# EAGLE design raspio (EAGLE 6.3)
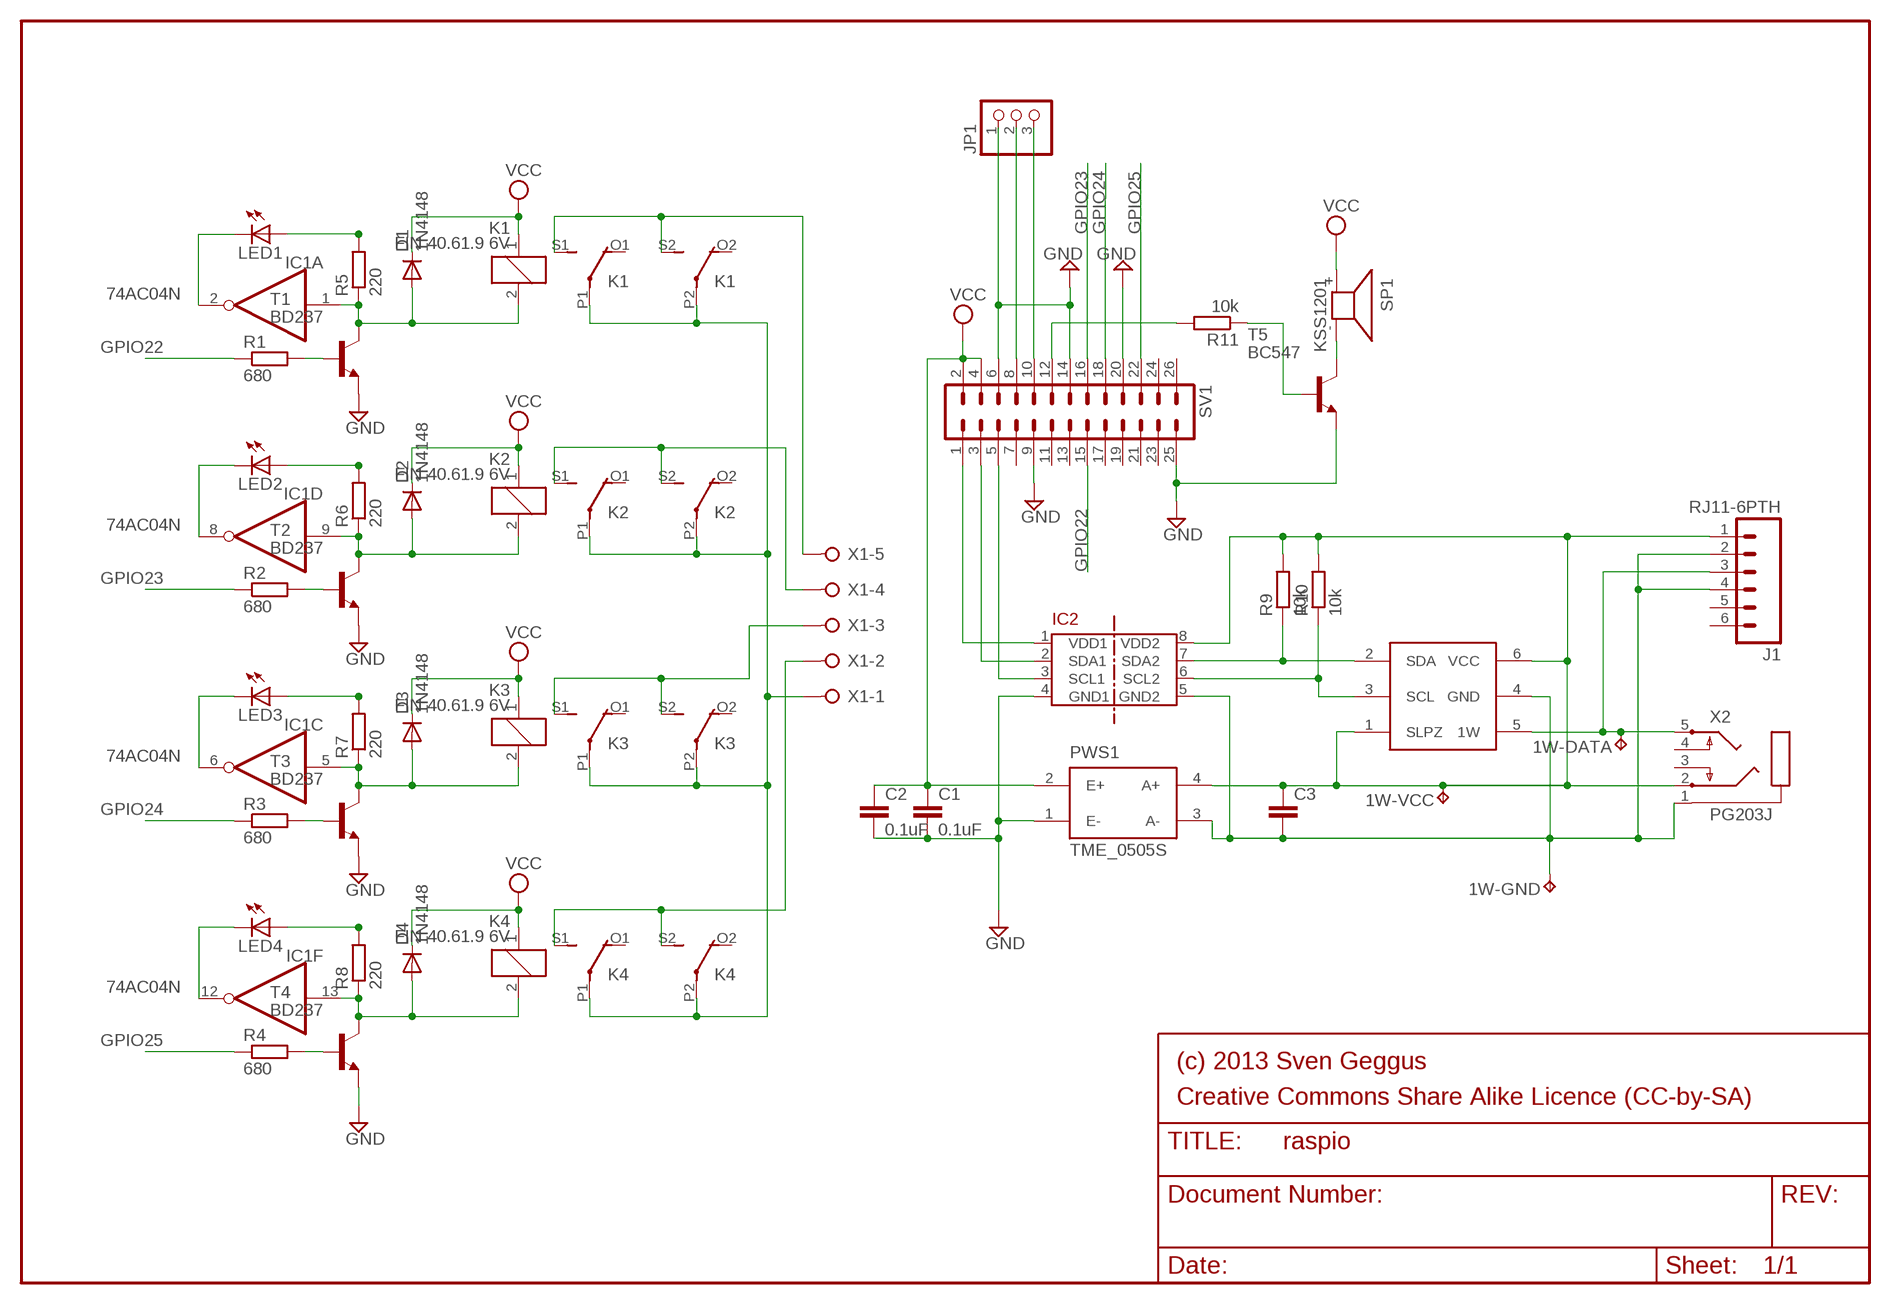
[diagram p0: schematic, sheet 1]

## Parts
1W-DATA  TPPAD1-13  [P1-13]
1W-GND  TPPAD1-13  [P1-13]
1W-VCC  TPPAD1-13  [P1-13]
C1  0.1uF  C-EU025-024X044  [C025-024X044]
C2  0.1uF  C-EU025-024X044  [C025-024X044]
C3  C-EU025-024X044  [C025-024X044]
D1  1N4148  [DO35-10]
D2  1N4148  [DO35-10]
D3  1N4148  [DO35-10]
D4  1N4148  [DO35-10]
IC1  74AC04N  [DIL14]
IC2  ADUM1250  [SO08]
IC3  DS2483  [TSOT23]
J1  RJ11-6PTH  [RJ11-6]
JP1  PINHD-1X3  [1X03]
K1  FIN 40.61.9 6V  4052  [F4052]
K2  FIN 40.61.9 6V  4052  [F4052]
K3  FIN 40.61.9 6V  4052  [F4052]
K4  FIN 40.61.9 6V  4052  [F4052]
LED1  LED5MM  [LED5MM]
LED2  LED5MM  [LED5MM]
LED3  LED5MM  [LED5MM]
LED4  LED5MM  [LED5MM]
PWS1  TME_0505S  [TMEXXXXS]
R1  680  R-EU_0207/10  [0207/10]
R2  680  R-EU_0207/10  [0207/10]
R3  680  R-EU_0207/10  [0207/10]
R4  680  R-EU_0207/10  [0207/10]
R5  220  R-EU_0207/10  [0207/10]
R6  220  R-EU_0207/10  [0207/10]
R7  220  R-EU_0207/10  [0207/10]
R8  220  R-EU_0207/10  [0207/10]
R9  10k  R-EU_0207/10  [0207/10]
R10  10k  R-EU_0207/10  [0207/10]
R11  10k  R-EU_0207/10  [0207/10]
SP1  KSS1201  [KSS1201]
SV1  ML26  [ML26]
T1  BD237  [TO126V]
T2  BD237  [TO126V]
T3  BD237  [TO126V]
T4  BD237  [TO126V]
T5  BC547  [TO92]
X1  W237-05P  [W237-5P]
X2  PG203J  [PG203J]

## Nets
GND: C1.2 C2.2 IC2.4(GND1) JP1.1 PWS1.1(E-) SV1.6 SV1.9 SV1.14 SV1.20 SV1.25 T1.1(E) T2.1(E) T3.1(E) T4.1(E) T5.1(E)
GPIO22: R1.1 SV1.15
GPIO23: R2.1 SV1.16
GPIO24: R3.1 SV1.18
GPIO25: R4.1 SV1.22
L: K3.S1(2:S) K3.S2(3:S) X1.3
N$1: K1.P1(2:P) K1.P2(3:P) K2.P1(2:P) K2.P2(3:P) K3.P1(2:P) K3.P2(3:P) K4.P1(2:P) K4.P2(3:P) X1.1
N$2: R1.2 T1.3(B)
N$3: IC1.2(A:O) LED1.K(C)
N$4: D2.A IC1.9(D:I) K2.2 R6.1 T2.2(C)
N$5: R11.2 SV1.12
N$6: R11.1 T5.2(B)
N$7: R2.2 T2.3(B)
N$8: D3.A IC1.5(C:I) K3.2 R7.1 T3.2(C)
N$9: K1.S1(2:S) K1.S2(3:S) X1.5
N$10: K2.S1(2:S) K2.S2(3:S) X1.4
N$11: R3.2 T3.3(B)
N$12: D4.A IC1.13(F:I) K4.2 R8.1 T4.2(C)
N$13: K4.S1(2:S) K4.S2(3:S) X1.2
N$14: SP1.- T5.3(C)
N$15: R4.2 T4.3(B)
N$16: D1.A IC1.1(A:I) K1.2 R5.1 T1.2(C)
N$18: IC1.8(D:O) LED2.K(C)
N$19: IC1.6(C:O) LED3.K(C)
N$20: IC1.12(F:O) LED4.K(C)
N$21: LED1.A R5.2
N$22: LED2.A R6.2
N$23: LED3.A R7.2
N$24: LED4.A R8.2
OW: 1W-DATA.TP IC3.5(1W) J1.3 X2.5
OWGND: 1W-GND.TP C3.2 IC2.5(GND2) IC3.4(GND) J1.2 J1.4 PWS1.3(A-) X2.1
OWSCL: IC2.6(SCL2) IC3.3(SCL) R10.1
OWSDA: IC2.7(SDA2) IC3.2(SDA) R9.1
OWVCC: 1W-VCC.TP C3.1 IC2.8(VDD2) IC3.1(SLPZ) IC3.6(VCC) J1.1 PWS1.4(A+) R9.2 R10.2 X2.2
RXD: JP1.3 SV1.10
SCL: IC2.3(SCL1) SV1.5
SDA: IC2.2(SDA1) SV1.3
TXD: JP1.2 SV1.8
VCC: C1.1 C2.1 D1.C D2.C D3.C D4.C K1.1 K2.1 K3.1 K4.1 PWS1.2(E+) SP1.+ SV1.2 SV1.4
VDD: IC2.1(VDD1) SV1.1
Unconnected: IC1.3(B:I) IC1.4(B:O) IC1.10(E:O) IC1.11(E:I) J1.5 J1.6 K1.O1(2:O) K1.O2(3:O) K2.O1(2:O) K2.O2(3:O) K3.O1(2:O) K3.O2(3:O) K4.O1(2:O) K4.O2(3:O) SV1.7 SV1.11 SV1.13 SV1.17 SV1.19 SV1.21 SV1.23 SV1.24 SV1.26 X2.3 X2.4

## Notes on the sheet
- (c) 2013 Sven Geggus
- Creative Commons Share Alike Licence (CC-by-SA)

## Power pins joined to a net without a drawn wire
GND: IC1.7(P:GND)
VCC: IC1.14(P:VCC)

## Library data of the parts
1W-DATA 1W-GND 1W-VCC = testpad:TP: Test pad
C1-C3 = rcl:C-EU: CAPACITOR, European symbol
D1-D4 = diode:1N4148: DIODE
IC1 = 74xx-eu:74*04: Hex INVERTER
IC2 = Bus-isolators:ADUM1250
IC3 = ds2483:DS2483: Single-Channel 1-Wire Master with Adjustable Timing and Sleep Mode
J1 = SparkFun-Connectors:RJ11-6: RJ11 Jack Simple 6 pin RJ11 jack. Commonly found on CAT3 devices and Microchip programmers. SKU: PRT-00132
JP1 = pinhead:PINHD-1X3: PIN HEADER
K1-K4 = relay:4052: RELAY 2 x switch, Finder
LED1-LED4 = led:LED: LED
PWS1 = traco-electronic:TME_*S: DC/DC Konverter 1 Watt Source: http://www.tracopower.com/datasheet_g/tme-d.pdf; MPN: TME 0505S; OC_FARNELL: 1007538; OC_NEWARK: 51R5321
R1-R11 = resistor:R-EU_: RESISTOR, European symbol
SP1 = buzzer:KSS1201: SPEAKER; OC_FARNELL: unknown; OC_NEWARK: unknown
SV1 = con-ml:ML26: HARTING; OC_FARNELL: unknown; OC_NEWARK: unknown
T1-T4 = sven-misc:BD237: NPN Transistor
T5 = transistor:BC547: NPN TRANSISTOR
X1 = con-wago-508:W237-05P: WAGO SREW CLAMP; OC_FARNELL: unknown; OC_NEWARK: unknown
X2 = con-hirschmann:PG203J: MIC/HEADPHONE JACK KS-S stereo microphone/headphone jack PG203JN (Schukat); OC_FARNELL: unknown; OC_NEWARK: unknown

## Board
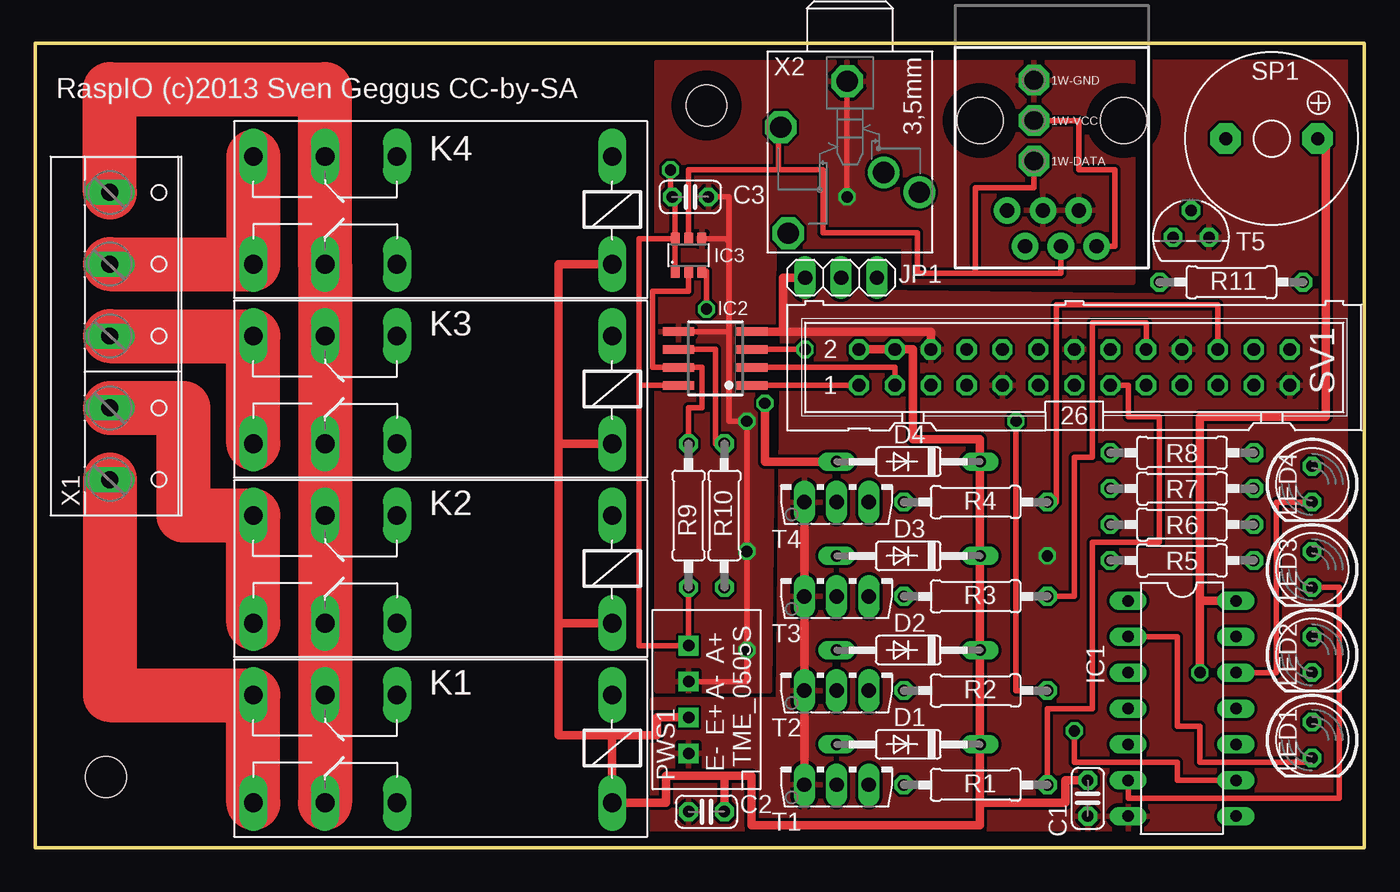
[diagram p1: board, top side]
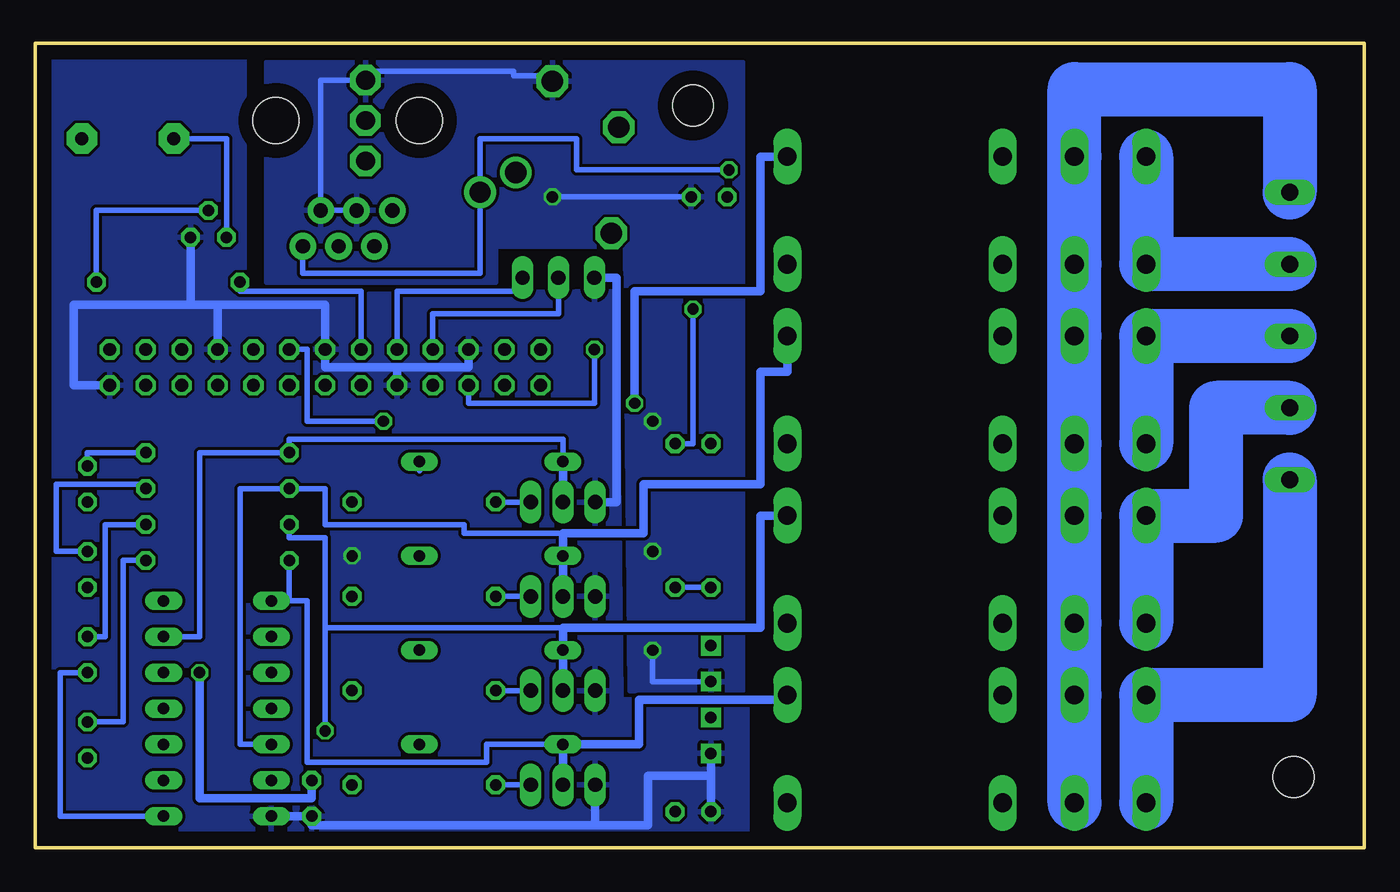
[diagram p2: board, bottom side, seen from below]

Size 94.05 x 56.92 mm. Coordinates in mm from the lower left corner, seen from the top.
Outline: 0,0 94.05,0 94.05,56.92 0,56.92 0,0
Copper layers (1*16): Top 0.035mm / dielectric 1.5mm / Bottom 0.035mm
Design rules "default": minimum track width 10mil, minimum drill 24mil, track to track 8mil, track to pad 8mil, pad to pad 8mil, via to via 8mil, smd to smd 8mil, copper to edge 40mil, drill to drill 8mil, minimum pad ring 10mil, minimum via ring 8mil, stop-mask expansion 4mil, vias tented up to drill 0mil, thermal gap 10mil
Holes 2.9 mm at 47.5,52.5 5,5

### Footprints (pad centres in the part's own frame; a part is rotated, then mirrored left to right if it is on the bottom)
P1-13 = drill 1.321 pad 2.159 octagon: TP 0,0
C025-024X044 = drill 0.813 octagon: 1 -1.27,0; 2 1.27,0
DO35-10 = drill 0.813 long: A 5.08,0; C -5.08,0
DIL14 = drill 0.813 long: 1 -7.62,-3.81; 2 -5.08,-3.81; 3 -2.54,-3.81; 4 0,-3.81; 5 2.54,-3.81; 6 5.08,-3.81; 7 7.62,-3.81; 8 7.62,3.81; 9 5.08,3.81; 10 2.54,3.81; 11 0,3.81; 12 -2.54,3.81; 13 -5.08,3.81; 14 -7.62,3.81
SO08 = smd 0.6 x 2.2: 1 -1.905,-2.6; 2 -0.635,-2.6; 3 0.635,-2.6; 4 1.905,-2.6; 5 1.905,2.6; 6 0.635,2.6; 7 -0.635,2.6; 8 -1.905,2.6
TSOT23 = smd 0.6 x 0.9: 1 -0.95,-1.15; 2 0,-1.15; 3 0.95,-1.15; 4 0.95,1.15; 5 0,1.15; 6 -0.95,1.15
RJ11-6 = drill 1.016 pad 1.88: 1 1.905,8.89; 2 3.175,6.35; 3 4.445,8.89; 4 5.715,6.35; 5 6.985,8.89; 6 8.255,6.35 | hole 3.251: 0,0; 10.16,0
1X03 = drill 1.016 long: 1 -2.54,0; 2 0,0; 3 2.54,0
F4052 = drill 1.321 long: 1 -3.81,3.81; 2 -3.81,-3.81; O1 11.43,-3.81; O2 11.43,3.81; P1 16.51,-3.81; P2 16.51,3.81; S1 21.59,-3.81; S2 21.59,3.81
LED5MM = drill 0.813 octagon: A -1.27,0; K 1.27,0
TMEXXXXS = drill 0.813 pad 1.397 square: 1 -3.81,1.27; 2 -1.27,1.27; 3 1.27,1.27; 4 3.81,1.27
0207/10 = drill 0.813 octagon: 1 -5.08,0; 2 5.08,0
KSS1201 = drill 0.914 pad 2.159 octagon: + 3.251,0; - -3.251,0
ML26 = drill 0.914 octagon: 1 -15.24,-1.27; 2 -15.24,1.27; 3 -12.7,-1.27; 4 -12.7,1.27; 5 -10.16,-1.27; 6 -10.16,1.27; 7 -7.62,-1.27; 8 -7.62,1.27; 9 -5.08,-1.27; 10 -5.08,1.27; 11 -2.54,-1.27; 12 -2.54,1.27; 13 0,-1.27; 14 0,1.27; 15 2.54,-1.27; 16 2.54,1.27; 17 5.08,-1.27; 18 5.08,1.27; 19 7.62,-1.27; 20 7.62,1.27; 21 10.16,-1.27; 22 10.16,1.27; 23 12.7,-1.27; 24 12.7,1.27; 25 15.24,-1.27; 26 15.24,1.27
TO126V = drill 1.016 long: 1 -2.286,-1.27; 2 0,-1.27; 3 2.286,-1.27
TO92 = drill 0.813 octagon: 1 1.27,0; 2 0,1.905; 3 -1.27,0
W237-5P = drill 1.194 long: 1 -10.16,-0.635; 2 -5.08,-0.635; 3 0,-0.635; 4 5.08,-0.635; 5 10.16,-0.635
PG203J = drill 1.499 octagon: 1 -5.004,-0.203; 4 5.74,-4.369; 5 -1.753,-4.902 | drill 1.499: 2 2.845,4.902; 3 1.448,2.388

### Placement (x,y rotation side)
1W-DATA  70.67,48.58 0 top
1W-GND  70.67,54.29 0 top
1W-VCC  70.67,51.44 0 top
C1  74.48,3.49 270 top
C2  47.5,2.54 180 top
C3  46.35,46.04 0 top
D1  61.78,7.3 180 top
D2  61.78,13.97 180 top
D3  61.78,20.64 180 top
D4  61.78,27.3 180 top
IC1  81.15,9.84 270 top
IC2  48.13,34.61 90 top
IC3  46.23,41.91 0 top
J1  77.03,51.44 180 top
JP1  57.02,40.32 0 top
K1  37.02,6.99 180 top
K2  37.02,19.68 180 top
K3  37.02,32.38 180 top
K4  37.02,45.09 180 top
LED1  90.36,7.62 270 top
LED2  90.36,13.65 270 top
LED3  90.36,19.68 270 top
LED4  90.36,25.72 270 top
PWS1  47.5,10.48 90 top
R1  66.55,4.45 180 top
R2  66.55,11.11 180 top
R3  66.55,17.78 180 top
R4  66.55,24.45 180 top
R5  81.15,20.32 0 top
R6  81.15,22.86 0 top
R7  81.15,25.4 0 top
R8  81.15,27.94 0 top
R9  46.23,23.5 270 top
R10  48.77,23.5 270 top
R11  84.64,40.01 180 top
SP1  87.5,50.16 0 top
SV1  73.53,33.97 0 top
T1  56.7,5.71 0 top
T2  56.7,12.38 0 top
T3  56.7,19.05 0 top
T4  56.7,25.72 0 top
T5  81.79,43.18 0 top
X1  5.91,36.2 270 top
X2  57.66,49.21 270 top

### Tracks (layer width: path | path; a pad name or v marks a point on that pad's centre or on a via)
GND  (via drill 0.8)
  Top 0.61: T4.1 T3.1 T2.1 T1.1 | SV1.6 63.37,36.51 52.9,36.51 | 52.9,36.51 IC2.4 | JP1.1 52.9,40.32 52.9,36.51
  Bottom 0.61: SV1.6 63.37,33.97 68.45,33.97 | SV1.9 68.45,33.97 | 68.45,33.97 73.53,33.97 SV1.14 73.53,38.42 81.15,38.42 | SV1.20 81.15,38.42 | 81.15,38.42 83.06,38.42 | 83.06,38.42 91.31,38.42 91.31,32.7 SV1.25 | T4.1 52.9,24.45 52.9,40.32 JP1.1 | T5.1 83.06,38.42 | IC1.7 C1.2 74.48,1.59 54.42,1.59 | T1.1 54.42,1.59 | 54.42,1.59 50.67,1.59 50.67,5.08 46.23,5.08 | C2.2 46.23,5.08 | 46.23,5.08 PWS1.1
  other vias: 71.63,20.64
  pour Bottom: 43.69,0 93.85,0 93.85,56.83 79.25,56.83 79.25,39.05 52.9,39.37 52.58,10.48 43.69,10.48
  pour Top: 43.69,0 93.85,0 93.85,56.83 79.25,56.83 79.25,39.05 52.9,39.37 52.58,10.48 43.69,10.48
GPIO22
  Top 0.406: SV1.15 77.34,32.7 77.34,30.48 79.56,30.48 79.56,21.59 74.8,21.59 74.8,9.84 71.63,9.84 R1.1
GPIO23  (via drill 0.8)
  Top 0.406: R2.1 69.41,11.11 v69.41,30.16
  Bottom 0.406: SV1.16 74.8,35.24 74.8,30.16 v69.41,30.16
GPIO24
  Top 0.406: SV1.18 78.61,37.15 74.8,37.15 74.8,27.62 73.53,27.62 73.53,17.78 R3.1
GPIO25
  Top 0.406: SV1.22 83.69,38.42 72.26,38.42 72.26,24.45 R4.1
L
  Top 3.81: X1.3 K3.S1 K3.S2
  Bottom 0.406: 15.43,36.51 K3.S1
  Bottom 3.81: K3.S2 K3.S1 X1.3
N$1
  Top 3.81: X1.1 5.27,53.66 20.51,53.66 K4.P1 K4.P2 K1.P2
  Bottom 3.81: K1.P2 K1.P1 K2.P2 K2.P1 K3.P2 K3.P1 K4.P2 K4.P1 20.51,53.66 5.27,53.66 X1.1
N$2
  Bottom 0.406: T1.3 R1.2
N$3
  Top 0.406: IC1.2 80.83,14.92 80.83,8.57 82.42,8.57 82.42,6.03 90.36,6.03 LED1.K
N$4  (via drill 0.8)
  Top 0.406: IC1.9 80.83,4.76 80.83,6.03 73.53,6.03 v73.53,8.26
  Bottom 0.406: R6.1 76.07,21.91 73.53,21.91 73.53,15.56 | v73.53,8.26 73.53,15.56 | 73.53,15.56 56.7,15.56
  Bottom 0.61: T2.2 D2.A 56.7,15.56 42.73,15.56 42.73,23.5 K2.2
N$5
  Bottom 0.406: SV1.12 70.99,39.37 79.56,39.37 R11.2
N$6
  Bottom 0.406: R11.1 89.72,45.09 T5.2
N$7
  Bottom 0.406: T2.3 R2.2
N$8
  Bottom 0.406: 56.7,22.23 63.69,22.23 63.69,22.86 73.53,22.86 73.53,25.4 R7.1 79.56,25.4 79.56,7.3 IC1.5
  Bottom 0.61: T3.2 D3.A 56.7,22.23 50.99,22.23 50.99,25.72 42.73,25.72 42.73,33.66 40.83,33.66 K3.2
N$9
  Top 3.81: K1.S2 K1.S1 5.27,10.79 X1.5
  Bottom 3.81: X1.5 5.27,10.79 K1.S1 K1.S2
N$10
  Top 3.81: X1.4 10.48,31.11 10.48,23.5 K2.S1 K2.S2
  Bottom 3.81: X1.4 10.48,31.11 10.48,23.5 K2.S1 K2.S2
N$11
  Bottom 0.406: T3.3 R3.2
N$12  (via drill 0.8)
  Top 0.61: v51.62,31.43 51.62,27.3 D4.A
  Bottom 0.406: D4.A 56.7,28.89 76.07,28.89 R8.1 82.42,27.94 82.42,14.92 IC1.13
  Bottom 0.61: T4.2 D4.A | K4.2 42.73,48.9 42.73,39.37 51.62,39.37 v51.62,31.43
N$13
  Top 3.81: X1.2 15.24,41.27 | K4.S2 15.24,41.27 | K4.S1 15.43,41.47 15.24,41.27
  Bottom 0.406: K4.S2 15.43,41.59
  Bottom 3.81: X1.2 K4.S2 K4.S1
N$14
  Bottom 0.406: SP1.- 80.52,50.16 T5.3
N$15
  Bottom 0.406: T4.3 R4.2
N$16
  Bottom 0.406: R5.1 76.07,17.46 | D1.A 62.1,7.3 62.1,6.03 74.8,6.03 74.8,17.46 76.07,17.46 | 76.07,17.46 IC1.1
  Bottom 0.61: T1.2 D1.A 51.31,7.3 51.31,10.48 40.83,10.48 K1.2
N$18
  Bottom 0.406: IC1.8 92.27,2.22 92.27,12.38 LED2.K
N$19
  Top 0.406: LED3.K 92.27,18.41 92.27,3.49 77.34,3.49 IC1.6
N$20
  Top 0.406: IC1.12 87.82,12.38 87.82,24.45 LED4.K
N$21
  Bottom 0.406: R5.2 87.82,20.32 87.82,8.89 LED1.A
N$22
  Bottom 0.406: LED2.A 89.09,14.92 89.09,22.86 R6.2
N$23
  Bottom 0.406: LED3.A 92.58,20.95 92.58,25.72 86.23,25.72 R7.2
N$24
  Bottom 0.406: LED4.A 90.36,27.94 R8.2
OW
  Top 0.406: IC3.5 46.23,47.94 52.58,47.94 | 52.58,47.94 52.58,50.97 X2.5 | 52.58,47.94 55.75,47.94 55.75,43.5 62.42,43.5 62.42,40.64 66.55,40.64 | 66.55,40.64 72.58,40.64 J1.3 | 1W-DATA.TP 70.67,46.67 66.55,46.67 66.55,40.64
OWGND  (via drill 0.8)
  Top 0.406: PWS1.3 50.35,11.75 v50.35,13.97 v50.35,20.95 v50.35,30.16 49.09,30.16 49.09,36.51 | IC2.5 49.09,36.51 | v57.45,46.04 X2.1 | 49.09,36.51 49.09,42.86 | 49.09,42.86 49.09,46.04 C3.2 | IC3.4 48.89,43.06 49.09,42.86
  Bottom 0.406: J1.4 J1.2 73.85,54.29 1W-GND.TP 70.67,54.93 60.2,54.93 60.2,54.61 57.45,54.61 X2.1 | PWS1.3 50.35,11.75 v50.35,13.97 | v57.45,46.04 C3.2
  pour Bottom: 44.01,55.56 77.66,55.56 77.66,40.01 61.47,40.01 61.47,42.55 52.26,42.55 51.94,11.11 44.01,11.11
  pour Top: 44.01,55.56 77.66,55.56 77.66,40.01 61.47,40.01 61.47,42.55 52.26,42.55 51.94,11.11 44.01,11.11
OWSCL  (via drill 0.8)
  Top 0.406: R10.1 48.13,28.57 48.13,35.24 IC2.6 | IC3.3 47.5,40.76 v47.5,38.1
  Bottom 0.406: v47.5,38.1 47.5,28.57 R10.1
OWSDA
  Top 0.406: IC3.2 46.23,39.37 43.69,39.37 43.69,33.97 IC2.7 47.18,33.97 47.18,31.11 46.23,31.11 R9.1
OWVCC  (via drill 0.8)
  Top 0.406: IC3.6 42.73,43.06 42.73,32.7 | 42.73,32.7 IC2.8 | IC3.1 IC3.6 | 42.73,32.7 42.73,14.29 PWS1.4 R9.2 | 1W-VCC.TP 73.85,51.44 73.85,47.94 76.39,47.94 76.39,42.55 J1.1 | IC3.6 45.27,46.04 C3.1 44.96,46.04 v44.96,47.94
  Bottom 0.406: R10.2 R9.2 | J1.1 75.12,40.64 62.56,40.64 X2.2 62.56,50.16 55.75,50.16 55.75,47.94 v44.96,47.94
RXD
  Bottom 0.406: SV1.10 68.45,39.37 59.56,39.37 JP1.3
SCL  (via drill 0.8)
  Top 0.406: IC2.3 v54.48,35.24
  Bottom 0.406: v54.48,35.24 54.48,31.43 63.37,31.43 SV1.5
SDA
  Top 0.406: IC2.2 60.83,33.97 SV1.3
TXD
  Bottom 0.406: SV1.8 65.91,37.78 57.02,37.78 JP1.2
VCC  (via drill 0.8)
  Top 0.61: SP1.+ 91.31,50.16 91.31,30.48 82.42,30.48 82.42,17.46 | SV1.2 SV1.4 62.1,35.24 62.1,28.89 66.86,28.89 D4.C D3.C D2.C D1.C | 40.83,7.94 K1.1 44.64,3.17 44.64,5.08 48.77,5.08 | 37.02,15.88 37.02,7.94 40.83,7.94 | 40.83,7.94 44.01,7.94 44.01,9.21 PWS1.2 | K2.1 37.02,15.88 | 37.02,15.88 37.02,28.57 | K3.1 37.02,28.57 | 37.02,28.57 37.02,41.27 K4.1 | D1.C 66.86,1.59 50.67,1.59 50.67,5.08 48.77,5.08 | 48.77,5.08 C2.1 | 82.42,17.46 IC1.14 | D1.C 66.86,3.17 72.9,3.17 72.9,4.76 C1.1 | 82.42,17.46 v82.42,12.38
  Bottom 0.406: 66.86,26.67 D4.C
  Bottom 0.61: v82.42,12.38 82.42,3.49 74.48,3.49 C1.1
VDD
  Top 0.406: SV1.1 IC2.1

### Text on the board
tNames: RaspIO (c)2013 Sven Geggus CC-by-SA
